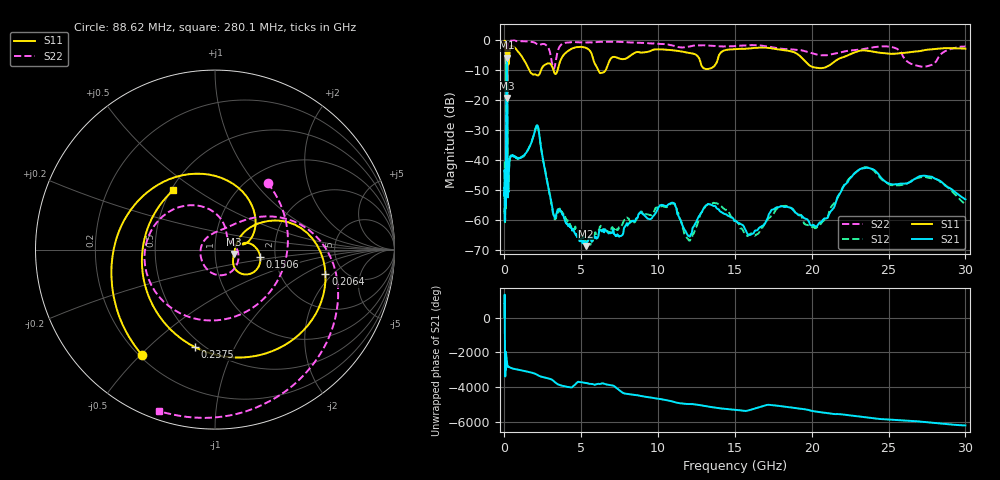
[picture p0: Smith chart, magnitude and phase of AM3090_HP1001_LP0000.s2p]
! Date/Time: Thu, Feb 28, 2019 2:02 PM
! Network Analyzer: Agilent Technologies E8364B Rev: A.07.50.67
! Sweep from 0.010 to 30.000 GHz, 1601 Points, Sweep Type: LOG
! Power Supply: 5.023 V, 0.002 A
# Hz S DB R 50
!freq MagS11 AngS11 MagS21 AngS21 MagS12 AngS12 MagS22 AngS22
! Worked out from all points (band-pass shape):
!   1601 points, 10 MHz to 30 GHz, reference 50 ohm
!   highest |S21| = -5.84 dB at 144 MHz (marker M1); lowest = -68.6 dB at 5.285 GHz (marker M2)
!   |S21| within 3 dB of the highest: 122.6 MHz to 177.1 MHz (54.53 MHz wide, 36.4 % of centre)
!   lowest |S11| = -19.3 dB at 179.4 MHz (marker M3), VSWR 1.24, Z = 61.7 - j2.99 ohm
!   |S11| at or under -10 dB: 1.605 GHz to 2.382 GHz (777.7 MHz wide, 39 % of centre); 3.186 GHz to 3.461 GHz (274.6 MHz wide, 8.26 % of centre); 6.099 GHz to 6.59 GHz (491.1 MHz wide, 7.74 % of centre)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
!   |S22| runs from -22.2 to -0.1 dB; largest |S21 - S12| = 0.014
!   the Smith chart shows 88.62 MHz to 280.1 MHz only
!   S11 on the Smith chart (normalised r, x): 88.62 MHz: 0.21, -0.50; 150.6 MHz: 1.67, -0.15; 206.4 MHz: 3.63, -1.62; 237.5 MHz: 0.45, -0.71; 280.1 MHz: 0.51, +0.41
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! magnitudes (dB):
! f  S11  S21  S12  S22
! 10 MHz  -0.3  -43.9  -40.4  -0.5
! 38.04 MHz  -0.5  -57.7  -60.3  -1.2
! 50.6 MHz  -0.8  -50.2  -49.4  -1.4
! 88.62 MHz  -2.9  -52.7  -52.4  -6.5
! 118.5 MHz  -8.9  -11.5  -11.5  -10.2
! 144 MHz  -13.2  -5.8  -5.8  -17.8
! 144.7 MHz  -13.0  -5.8  -5.8  -17.6
! 150.6 MHz  -11.9  -5.9  -5.9  -16.4
! 179.4 MHz  -19.3  -9.7  -9.7  -18.4
! 206.4 MHz  -4.0  -47.5  -46.8  -2.5
! 237.5 MHz  -5.1  -51.4  -50.8  -0.8
! 280.1 MHz  -7.9  -45.6  -45.7  -0.4
! 550.5 MHz  -2.1  -38.6  -38.4  -0.2
! 2.084 GHz  -11.7  -28.7  -28.6  -1.2
! 3.22 GHz  -10.6  -58.6  -58.9  -9.6
! 5.285 GHz  -2.6  -68.6  -66.9  -0.8
! 7.926 GHz  -6.1  -61.6  -59.5  -0.7
! 10.65 GHz  -3.3  -54.8  -55.2  -1.5
! 12.01 GHz  -4.3  -65.4  -66.8  -2.2
! 20.2 GHz  -9.1  -62.0  -62.7  -4.6
! 23.36 GHz  -3.4  -42.7  -42.6  -3.0
! 30 GHz  -2.9  -53.1  -54.7  -2.2
